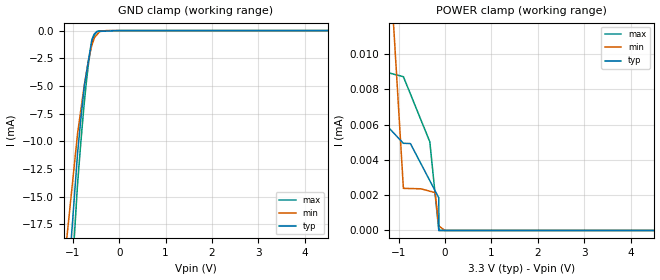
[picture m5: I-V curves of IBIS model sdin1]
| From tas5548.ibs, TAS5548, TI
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|   sdin1 Model
[Model]   sdin1
Model_type   Input
Vinl = 0.8
Vinh = 2.0
|   typ   min   max
|   (nom PVT)   (fast PVT)   (slow PVT)
|C_comp from frequency sweep method (F=25MHz)
|Average
|C_comp   5.385e-12   5.278e-12   5.492e-12
|C_comp from LC tank measurement(L=1nH)
|Average
|Resonant Frequency(Hz)   3.670e+09   4.640e+09   3.180e+09
C_comp   1.883e-12   1.178e-12   2.507e-12
| Where nom  PVT is Nominal Process, 3.3V, 27C
|   Fast PVT is Strong Process,  3.6V, 0C
|   Slow PVT is Weak Process,   3V, 125C
[Voltage Range]   3.3   3   3.6
|Ambient Temperature   27   125   0
|Junction Temperature
[Temperature Range]   27   125   0
[Power Clamp Reference]   3.3   3   3.6
[GND Clamp Reference]   0   0   0
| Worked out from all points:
|   GND clamp passes 1 mA (typ) near -0.60 V on its own axis
|   POWER clamp passes 1 mA (typ) near -3.28 V on its own axis
[GND Clamp]
|   Voltage   I(typ)   I(min)   I(max)
-3.3V     -1.926A    -1.648A    -2.038A
-1.58V    -50.02mA   -37.1mA    -60.13mA
-897.6mV  -11.09mA   -9.308mA   -13.88mA
-831.6mV  -8.188mA   -7.308mA   -10.33mA
-745.8mV  -4.835mA   -4.756mA   -6.256mA
-666mV    -2.783mA   -2.777mA   -3.13mA
-590.7mV  -846.8uA   -1.364mA   -1.192mA
-532.8mV  -295.9uA   -648.8uA   -372.1uA
-481.8mV  -81.38uA   -386.4uA   -111.9uA
-420mV    -70.87uA   -83.04uA   -28.92uA
-285mV    -47.91uA   -3.547uA   -15.31uA
6.6V      0A         0A         0A
[POWER Clamp]
|   Voltage   I(typ)   I(min)   I(max)
-3.3V     1.043mA    5.986mA    1.052mA
-2.262V   46.15uA    205.9uA    34.83uA
-2.059V   8.187uA    121.1uA    9.526uA
-1.878V   7.681uA    45.37uA    9.4uA
-896.4mV  4.943uA    2.387uA    8.718uA
-745.8mV  4.928uA    2.378uA    7.741uA
-327.6mV  2.826uA    2.227uA    5.03uA
-213mV    2.25uA     2.147uA    2.067uA
-133.2mV  1.849uA    282.3nA    0A
-132mV    0A         254.3nA    0A
-3.3mV    0A         0A         0A
6.6V      0A         0A         0A
